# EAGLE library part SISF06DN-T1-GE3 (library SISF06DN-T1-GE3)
1-MOSFET Dual N-Ch 30V(S1-S2) Source: Datasheet
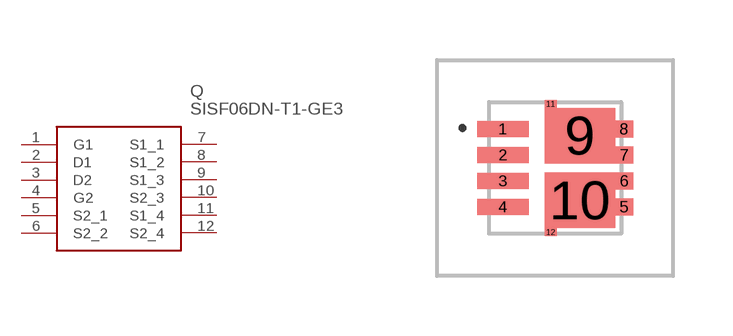
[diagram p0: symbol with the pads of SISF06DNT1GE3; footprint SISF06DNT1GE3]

Designator prefix Q

## SISF06DN-T1-GE3 (Description: 1-MOSFET Dual N-Ch 30V(S1-S2); Height: 0.8mm; Manufacturer_Name: Vishay; Manufacturer_Part_Number: SISF06DN-T1-GE3; Mouser_Part_Number: 78-SISF06DN-T1-GE3; Mouser_Price-Stock: https://www.mouser.co.uk/ProductDetail/Vishay-Siliconix/SISF06DN-T1-GE3?qs=vmHwEFxEFR9s9AAsXqpgFQ%3D%3D)  [SISF06DNT1GE3]
1  G1
2  D1
3  D2
4  G2
5  S2_1
6  S2_2
7  S1_1
8  S1_2
9  S1_3
10  S2_3
11  S1_4
12  S2_4

## Footprint SISF06DNT1GE3 (pad centres in mm)
SISF06DN-T1-GE3-3
smd 1.29 x 0.4: 1 -1.342,0.975; 2 -1.342,0.325; 3 -1.342,-0.325; 4 -1.342,-0.975
smd 0.45 x 0.42: 5 1.688,-0.975; 6 1.688,-0.325; 7 1.688,0.325; 8 1.688,0.975
smd 1.76 x 1.39: 9 0.583,0.81; 10 0.583,-0.81
smd 0.3 x 0.2: 11 -0.147,1.605; 12 -0.147,-1.605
